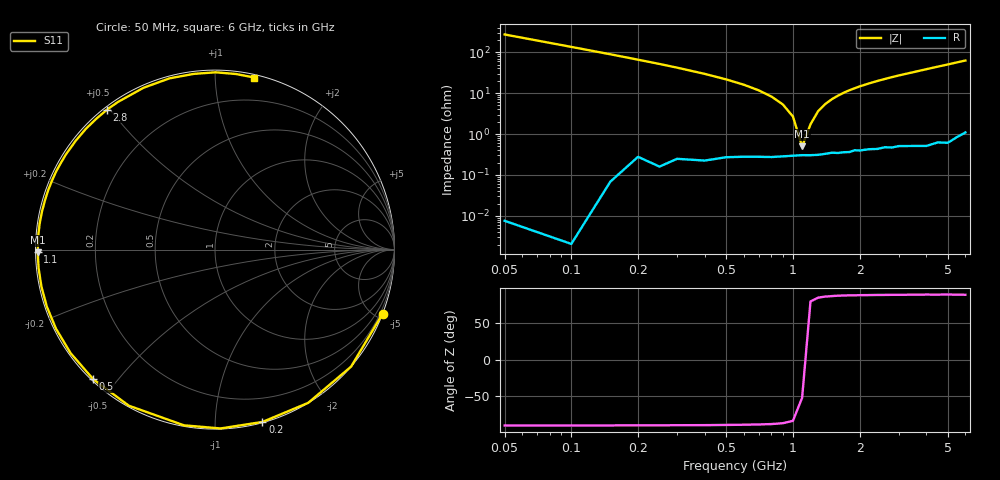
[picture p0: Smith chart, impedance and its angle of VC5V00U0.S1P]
! Infineon Technologies  Discrete & RF Semiconductors
! BBY 56-03
! Si Tuning Diode in SOD323
! VR = 5 V
! S-Parameters:  June  1999
# GHz  S  MA  R  50
!  f  S11
! GHz  MAG  ANG
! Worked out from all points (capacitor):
!   34 points, 50 MHz to 6 GHz, reference 50 ohm
!   read as one part to ground: C = 11.7 pF near 50 MHz
!   lowest |Z| = 497 mohm at 1.1 GHz (marker M1)
!   series resonance near 1.119 GHz, so ESL is about 1.7 nH
!   S11 on the Smith chart (normalised r, x): 50 MHz: 0.00, -5.42; 200 MHz: 0.01, -1.31; 500 MHz: 0.01, -0.43; 1.1 GHz: 0.01, -0.01; 2.8 GHz: 0.01, +0.49; 6 GHz: 0.02, +1.25
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0.05  1 -20.9
0.1  1 -40.7
0.15  0.9993 -58.7
0.2  0.9959 -74.6
0.25  0.9969 -88.2
0.3  0.9942 -100.0
0.4  0.9933 -118.9
0.5  0.9909 -133.2
0.6  0.9899 -144.4
0.7  0.9895 -153.6
0.8  0.9894 -161.3
0.9  0.9888 -167.9
1  0.9883 -173.9
1.1  0.9879 -179.1
1.3  0.9877 171.7
1.4  0.9871 167.6
1.6  0.9867 160.2
1.8  0.9863 153.5
2  0.9855 147.5
2.4  0.9851 136.9
2.8  0.985 127.6
3  0.9844 123.3
3.5  0.9857 113.8
4  0.9872 104.9
4.5  0.9861 96.9
5  0.9879 89.8
5.5  0.9853 83.1
6  0.9831 77.2
